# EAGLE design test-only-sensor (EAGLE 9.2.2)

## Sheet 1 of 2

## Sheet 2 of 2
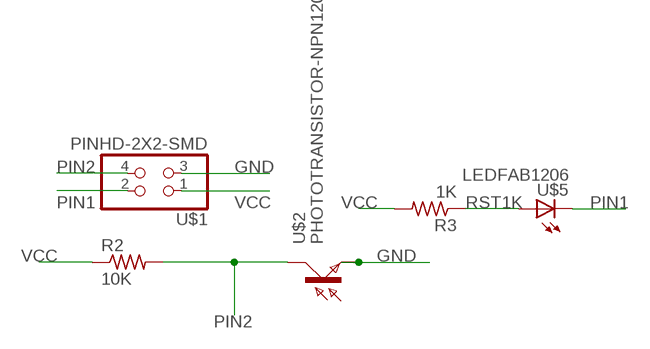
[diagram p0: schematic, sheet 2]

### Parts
R2  10K  RES-US1206FAB  [R1206FAB]
R3  1K  RES-US1206FAB  [R1206FAB]
U$1  PINHD-2X2-SMD  [2X02SMD]
U$2  PHOTOTRANSISTOR-NPN1206  [OP1206]
U$5  LEDFAB1206  [LED1206FAB]

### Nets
GND: U$1.3 U$2.EMITTER(E)
PIN1: U$1.2 U$5.2(C)
PIN2: R2.2 U$1.4 U$2.COLLECTOR(C)
RST1K: R3.1 U$5.1(A)
VCC: R2.1 R3.2 U$1.1

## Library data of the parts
R2 R3 = fab:RES-US: Resistor (US Symbol)
U$1 = fab:PINHD-2X2-SMD
U$2 = fab:PHOTOTRANSISTOR-NPN
U$5 = fab:LED: LED

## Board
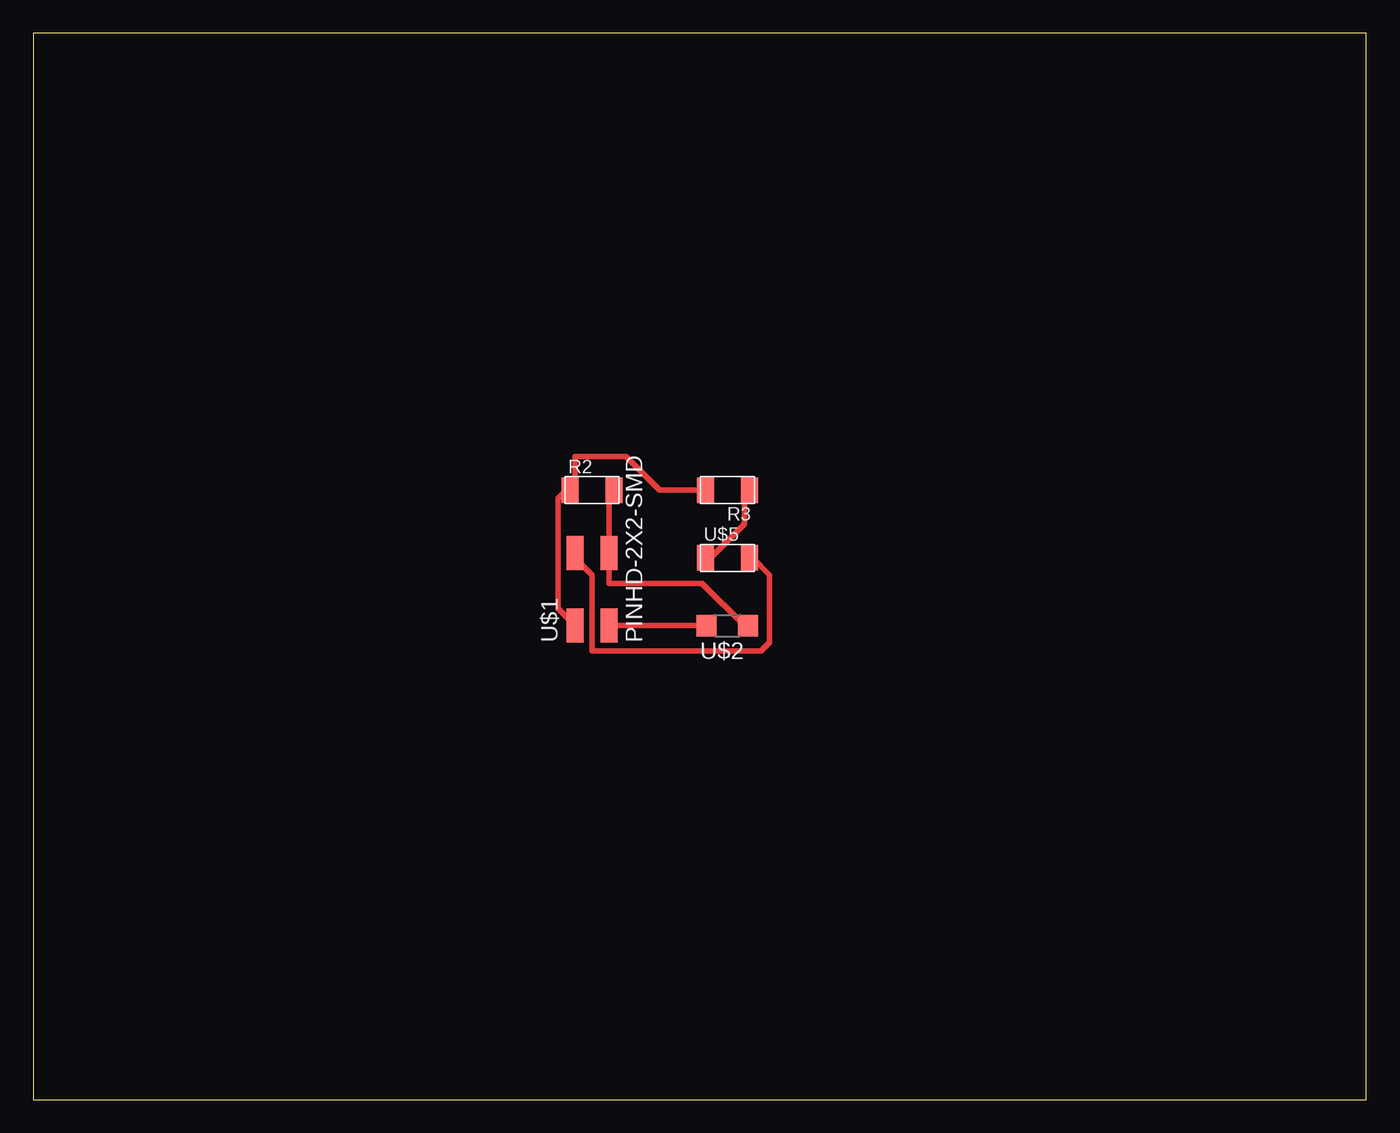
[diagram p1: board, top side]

Size 100 x 80 mm. Coordinates in mm from the lower left corner, seen from the top.
Outline: 0,0 100,0 100,80 0,80 0,0
Copper layers (1*16): Top 0.035mm / dielectric 1.5mm / Bottom 0.035mm
Design rules "default *": minimum track width 16mil, minimum drill 0.35mm, track to track 16mil, track to pad 16mil, pad to pad 16mil, via to via 16mil, smd to smd 16mil, copper to edge 40mil, drill to drill 16mil, minimum pad ring 10mil, minimum via ring 8mil, stop-mask expansion 4mil, vias tented up to drill 0mil, thermal gap 10mil

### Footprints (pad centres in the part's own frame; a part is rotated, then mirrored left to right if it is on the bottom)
R1206FAB = smd 1.27 x 1.905: 1 -1.651,0; 2 1.651,0
2X02SMD = smd 2.54 x 1.27: 1 -2.54,1.27; 2 2.92,1.27; 3 -2.54,-1.27; 4 2.92,-1.27
OP1206 = smd 1.5 x 1.6: COLLECTOR -1.55,0; EMITTER 1.55,0
LED1206FAB = smd 1.27 x 1.905: 1 -1.651,0; 2 1.651,0

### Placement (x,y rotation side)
R2  41.91,45.72 0 top
R3  52.07,45.72 180 top
U$1  41.91,38.1 90 top
U$2  52.07,35.56 180 top
U$5  52.07,40.64 0 top

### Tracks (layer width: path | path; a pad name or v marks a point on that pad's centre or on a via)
GND
  Top 0.406: U$1.3 U$2.EMITTER
PIN1
  Top 0.406: U$5.2 53.98,40.64 55.24,39.37 55.24,34.29 54.61,33.66 41.91,33.66 41.91,39.37 40.64,40.64 U$1.2
PIN2
  Top 0.406: R2.2 43.18,45.72 U$1.4 43.18,38.73 50.16,38.73 53.34,35.56 U$2.COLLECTOR
RST1K
  Top 0.406: U$5.1 50.8,40.64 53.34,43.18 53.34,45.72 R3.1
VCC
  Top 0.406: U$1.1 39.37,36.83 39.37,45.09 40.01,45.72 R2.1 | 50.16,45.72 R3.2 46.99,45.72 44.45,48.26 40.64,48.26 40.64,46.1 R2.1 | 40.64,45.72 R2.1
